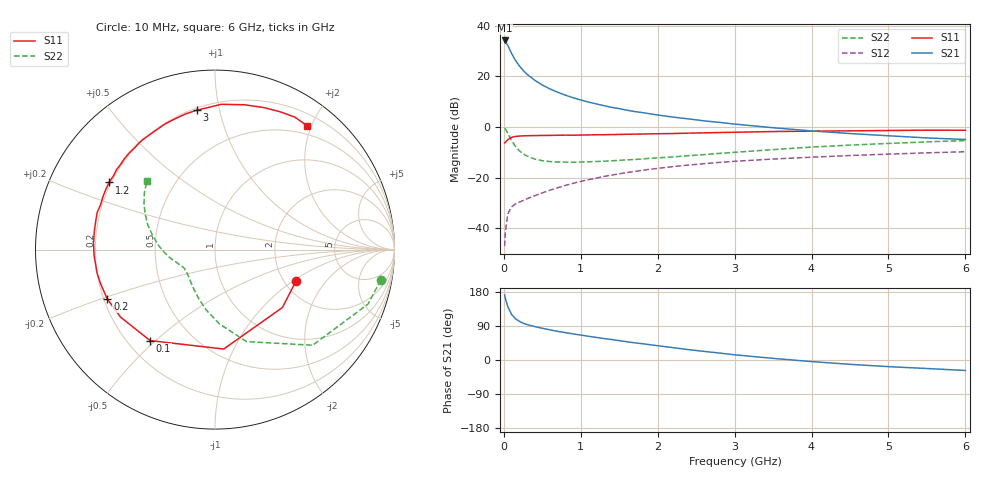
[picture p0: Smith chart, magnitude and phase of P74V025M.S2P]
! SIEMENS Small Signal Semiconductors
! BFP196
! Si NPN RF Bipolar Junction Transistor in SOT143
! VCE = 4 V  IC = 25 mA
! Common Emitter S-Parameters:  May  1996
# GHz  S  MA  R  50
!  f  S11  S21  S12  S22
! GHz  MAG  ANG  MAG  ANG  MAG  ANG  MAG  ANG
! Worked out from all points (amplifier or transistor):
!   36 points, 10 MHz to 6 GHz, reference 50 ohm
!   highest |S21| = 34.2 dB at 10 MHz (marker M1)
!   |S21| within 3 dB of that: start of sweep to 67.22 MHz
!   unconditionally stable (mu >= 1): 618.8 MHz to 3.42 GHz
!   at 250 MHz: K = 0.66, MSG = 25.7 dB, |S12| = -29.1 dB
!   at 1.4 GHz: K = 1.10, MAG = 11.5 dB, |S12| = -19.1 dB
!   at 6 GHz: K = 0.97, MSG = 2.4 dB, |S12| = -9.8 dB
!   S11 on the Smith chart (normalised r, x): 10 MHz: 2.31, -1.06; 100 MHz: 0.29, -0.48; 200 MHz: 0.21, -0.21; 1.2 GHz: 0.19, +0.28; 3 GHz: 0.21, +0.86; 6 GHz: 0.37, +1.94
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0.01  0.4843 -21.2  51.07 171.5  0.0044 84.1  0.9392 -10.4
0.02  0.4951 -40.7  48.86 162.1  0.0084 75.2  0.9049 -19.6
0.05  0.5562 -85.0  41 141.5  0.0187 59.3  0.7617 -44.4
0.1  0.6226 -125.5  28.46 120.5  0.0263 46.3  0.5416 -71.1
0.15  0.6471 -144.5  20.71 109.1  0.03 43.6  0.4133 -86.8
0.2  0.6598 -155.4  16.19 102.2  0.0326 42.9  0.3401 -98.2
0.25  0.6653 -163.3  13.08 97.3  0.0351 43.7  0.293 -107.2
0.3  0.67 -168.8  11.02 93.6  0.038 45.9  0.2661 -113.7
0.4  0.6745 -177.4  8.388 88.2  0.0436 48.8  0.2319 -124.3
0.5  0.6777 176.8  6.722 83.7  0.0497 51.7  0.2147 -132.0
0.6  0.6798 171.7  5.622 79.5  0.0562 53.1  0.2063 -137.3
0.7  0.683 166.7  4.837 75.5  0.0628 54.5  0.2024 -141.5
0.9  0.6845 158.7  3.769 68.9  0.0768 55.3  0.2 -147.9
1.1  0.6945 151.1  3.099 62.6  0.0906 55.0  0.2047 -152.1
1.2  0.6988 147.6  2.85 59.6  0.0973 54.8  0.207 -154.1
1.6  0.7155 134.7  2.137 48.2  0.1253 51.2  0.2235 -160.5
2.2  0.7399 117.4  1.561 32.6  0.164 44.5  0.2556 -169.8
3  0.7831 97.4  1.138 13.7  0.2093 34.1  0.3145 176.0
3.5  0.8102 87.5  0.962 4.3  0.2317 27.7  0.3558 167.4
4.5  0.8368 71.0  0.739 -11.4  0.2718 16.2  0.4369 153.0
5.5  0.8618 58.9  0.606 -22.5  0.3072 5.4  0.506 141.0
6  0.8597 53.2  0.564 -27.6  0.3234 -0.3  0.5366 135.0
